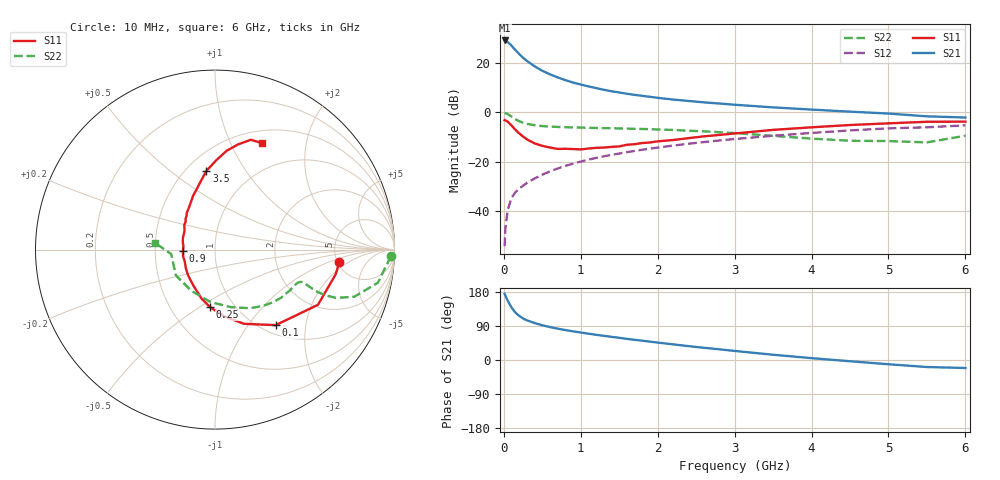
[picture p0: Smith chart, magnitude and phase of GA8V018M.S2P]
! Infineon Technologies  Discrete & RF Semiconductors
! BF775
! Si NPN RF Bipolar Junction Transistor in SOT23
! VCE = 8 V  IC = 18 mA
! Common Emitter S-Parameters:  May  1996
# GHz  S  MA  R  50
!  f  S11  S21  S12  S22
! GHz  MAG  ANG  MAG  ANG  MAG  ANG  MAG  ANG
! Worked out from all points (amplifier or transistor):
!   36 points, 10 MHz to 6 GHz, reference 50 ohm
!   highest |S21| = 29.3 dB at 10 MHz (marker M1)
!   |S21| within 3 dB of that: start of sweep to 124.8 MHz
!   unconditionally stable (mu >= 1): 462.4 MHz to 2.735 GHz
!   at 250 MHz: K = 0.80, MSG = 26.0 dB, |S12| = -29.8 dB
!   at 1.4 GHz: K = 1.10, MAG = 11.0 dB, |S12| = -17.3 dB
!   at 6 GHz: K = 0.90, MSG = 1.6 dB, |S12| = -5.3 dB
!   S11 on the Smith chart (normalised r, x): 10 MHz: 5.20, -1.39; 100 MHz: 1.15, -1.37; 250 MHz: 0.77, -0.55; 900 MHz: 0.70, -0.01; 3.5 GHz: 0.62, +0.68; 6 GHz: 0.64, +1.32
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0.01  0.6962 -5.7  29.04 174.6  0.0019 86.6  0.9808 -2.2
0.02  0.6862 -11.6  28.67 169.7  0.0043 83.9  0.9621 -4.8
0.05  0.651 -28.2  27.05 156.6  0.0103 79.1  0.9262 -11.5
0.1  0.54 -51.2  22.76 138.5  0.0183 70.2  0.8193 -18.7
0.15  0.4439 -68.7  18.53 125.1  0.0237 65.7  0.725 -21.8
0.2  0.3738 -82.5  15.37 116.3  0.0283 65.6  0.6609 -22.5
0.25  0.3219 -94.9  12.92 109.6  0.0322 65.6  0.6156 -22.4
0.3  0.2832 -105.3  11.12 104.6  0.0368 66.7  0.5843 -21.9
0.4  0.2338 -120.9  8.659 97.6  0.0452 67.5  0.5481 -21.0
0.5  0.2086 -135.6  7.016 91.6  0.054 69.0  0.5263 -20.6
0.6  0.1925 -147.7  5.939 86.9  0.0632 69.7  0.5147 -20.5
0.7  0.1807 -158.9  5.148 82.7  0.0721 69.9  0.5058 -20.9
0.8  0.1817 -167.8  4.523 79.0  0.0816 69.6  0.4994 -21.5
0.9  0.1796 -177.3  4.045 75.6  0.0906 69.4  0.494 -22.3
1.1  0.1839 167.1  3.379 69.5  0.1093 68.6  0.4855 -24.5
1.3  0.1927 155.7  2.88 63.8  0.1278 67.3  0.4788 -26.8
1.6  0.2193 141.3  2.392 55.7  0.1552 65.1  0.467 -31.2
2.2  0.274 122.2  1.824 41.3  0.2112 59.7  0.4386 -41.4
3.5  0.4409 96.3  1.264 13.9  0.3344 45.5  0.3329 -74.5
4.5  0.5532 83.4  1.035 -3.3  0.4299 33.0  0.2648 -119.8
5.5  0.6439 71.9  0.831 -18.5  0.4974 17.7  0.2452 -174.2
6  0.648 66.4  0.786 -21.1  0.5447 13.4  0.3352 173.7
